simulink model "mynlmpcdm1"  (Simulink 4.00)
settings: Solver=ode45  SolverMode=SingleTasking  StartTime=0.0  StopTime=4  MaxStep=0.2  RelTol=1e-3  AbsTol=1e-6
PreLoadFcn:
  | demo1dat
libraries: nlmpclib x1

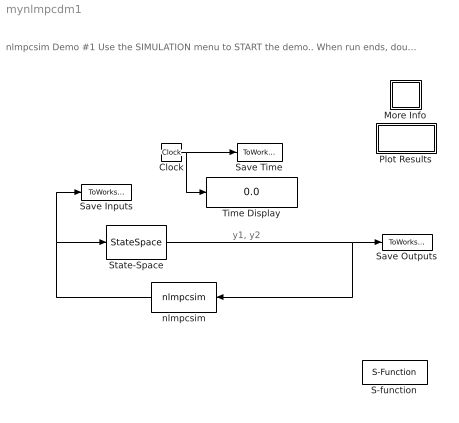
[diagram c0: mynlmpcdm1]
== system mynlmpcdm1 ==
  note: y1, y2
  note: nlmpcsim Demo #1 Use the SIMULATION menu to START the demo.. When run ends, double click on PLOT RESULTS. (Double click on the "?" for more info)
  Clock : Clock
  More Info : Subsystem
  Plot Results : Subsystem
  S-function : S-Function  FunctionName=mpcplant  PortCounts=[]  SFunctionModules=''
  Save Inputs : ToWorkspace  VariableName=u  SampleTime=0  SaveFormat=Array
  Save Outputs : ToWorkspace  VariableName=y  SampleTime=0  SaveFormat=Array
  Save Time : ToWorkspace  VariableName=t  SampleTime=0  SaveFormat=Array
  State-Space : StateSpace  A=eye(2)  B=eye(2)  C=eye(2)  D=eye(2)  X0=0  AbsoluteTolerance=auto  Realization=auto
  Time Display : Display
  nlmpcsim : nlmpclib/nlmpcsim  Orientation=left
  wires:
  State-Space/1 -> Save Outputs/1, nlmpcsim/1
  nlmpcsim/1 -> Save Inputs/1, State-Space/1
  Clock/1 -> Save Time/1, Time Display/1

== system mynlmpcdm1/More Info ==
  note: After the simulation ends, double-click on "Plot Results". Inputs and outputs will be plotted in a figure window using the MPC Tools "ploteach" command.
  note: Use the Simulation menu to Start the simulation.
  note: This demonstration shows how masked variables are specified for nlmpcsim. See the manual for details.

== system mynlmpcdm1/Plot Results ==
